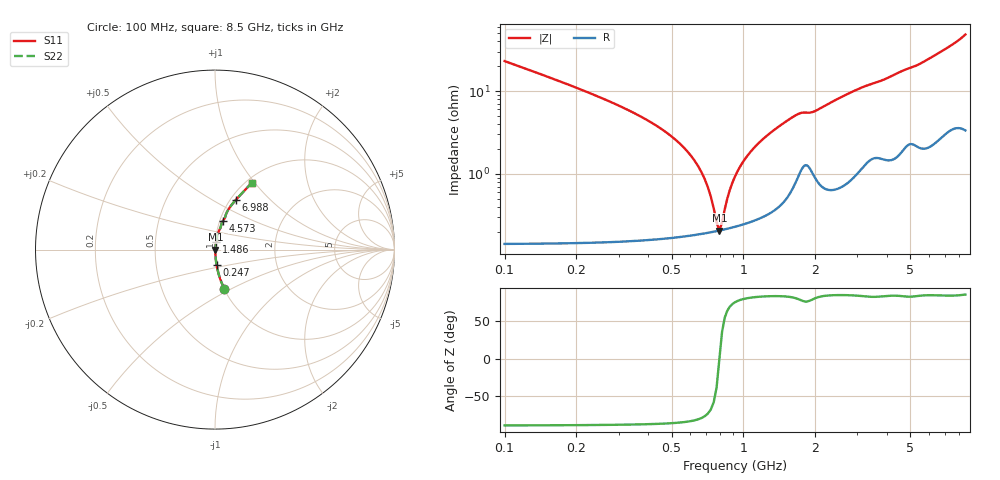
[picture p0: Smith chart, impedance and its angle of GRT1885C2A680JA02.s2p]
!Murata Part Number: GRT1885C2A680JA02
!These Parameters are Measured in Series Mode Connection
!Data Generated on Jun 19, 2026
!  o--ll--o
!Port1  Port2
!  o------o
!Operation Temp=25[degC], DC Bias Voltage=0[V]
!Freq. Start=100[MHz] Stop=9[GHz] 401[Steps]
# Hz S RI R 50
!Freq.(Hz) S11(Real) S11(Imag) S21(Real) S21(Imag) S12(Real) S12(Imag) S22(Real) S22(Imag)
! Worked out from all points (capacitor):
!   401 points, 100 MHz to 8.5 GHz, reference 50 ohm
!   read as one part in series: C = 68 pF near 142 MHz
!   lowest |Z| = 206 mohm at 793 MHz (marker M1)
!   series resonance near 793.3 MHz, so ESL is about 590 pH
!   S11 on the Smith chart (normalised r, x): 100 MHz: 1.00, -0.46; 247 MHz: 1.00, -0.17; 1.486 GHz: 1.01, +0.08; 4.573 GHz: 1.04, +0.34; 6.988 GHz: 1.06, +0.64; 8.5 GHz: 1.07, +0.96
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1e8  0.0516 -0.2182  0.9484 0.2182  0.9484 0.2182  0.0516 -0.2182
2.47e8  0.00872 -0.0847  0.9913 0.0847  0.9913 0.0847  0.00872 -0.0847
6.04e8  0.00206 -0.0163  0.9979 0.0163  0.9979 0.0163  0.00206 -0.0163
6.88e8  0.00197 -0.00844  0.998 0.00844  0.998 0.00844  0.00197 -0.00844
7.72e8  0.00203 -0.00161  0.998 0.00161  0.998 0.00161  0.00203 -0.00161
7.93e8  0.00206 -2.17e-05  0.9979 2.17e-05  0.9979 2.17e-05  0.00206 -2.17e-05
8.35e8  0.00214 0.00304  0.9979 -0.00304  0.9979 -0.00304  0.00214 0.00304
8.77e8  0.00224 0.00596  0.9978 -0.00596  0.9978 -0.00596  0.00224 0.00596
9.19e8  0.00235 0.00876  0.9976 -0.00876  0.9976 -0.00876  0.00235 0.00876
1.024e9  0.00273 0.0154  0.9973 -0.0154  0.9973 -0.0154  0.00273 0.0154
1.213e9  0.00371 0.0263  0.9963 -0.0263  0.9963 -0.0263  0.00371 0.0263
1.486e9  0.00634 0.041  0.9937 -0.041  0.9937 -0.041  0.00634 0.041
1.507e9  0.00667 0.0421  0.9933 -0.0421  0.9933 -0.0421  0.00667 0.0421
1.717e9  0.0126 0.0516  0.9874 -0.0516  0.9874 -0.0516  0.0126 0.0516
1.948e9  0.0129 0.0536  0.9871 -0.0536  0.9871 -0.0536  0.0129 0.0536
2.914e9  0.0188 0.0976  0.9812 -0.0976  0.9812 -0.0976  0.0188 0.0976
4.3e9  0.0383 0.1495  0.9617 -0.1495  0.9617 -0.1495  0.0383 0.1495
4.573e9  0.0449 0.1613  0.9551 -0.1613  0.9551 -0.1613  0.0449 0.1613
5.707e9  0.0658 0.2076  0.9342 -0.2076  0.9342 -0.2076  0.0658 0.2076
6.988e9  0.1143 0.2748  0.8857 -0.2748  0.8857 -0.2748  0.1143 0.2748
7.114e9  0.1203 0.2814  0.8797 -0.2814  0.8797 -0.2814  0.1203 0.2814
8.5e9  0.2053 0.3707  0.7947 -0.3707  0.7947 -0.3707  0.2053 0.3707
